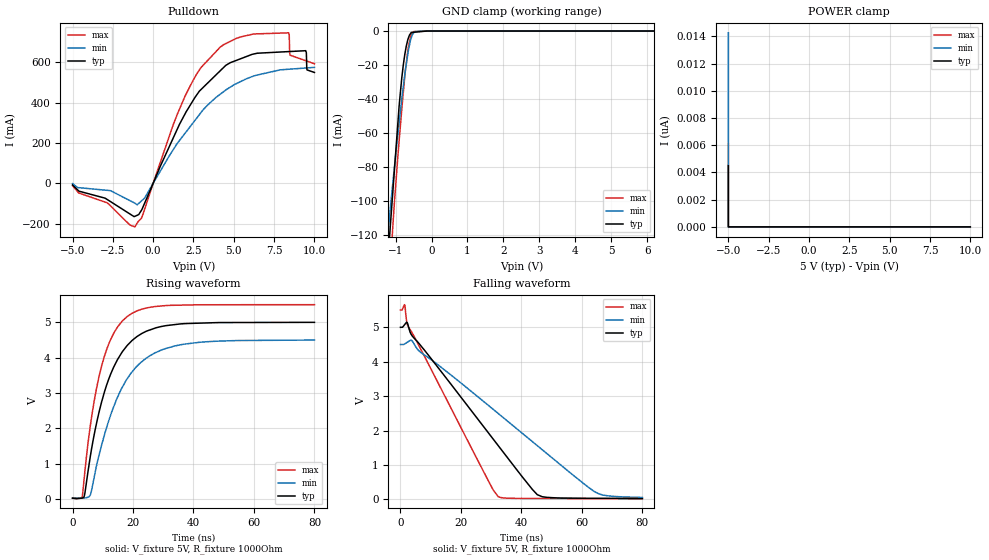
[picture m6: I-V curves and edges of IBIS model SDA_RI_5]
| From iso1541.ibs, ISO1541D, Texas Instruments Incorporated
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|   SDA Right 5V I/O Model
[Model]   SDA_RI_5
Model_type   I/O_open_drain
Polarity   Non-Inverting
Enable   Active-Low
Vinl = 1.35
Vinh = 3.85
Vmeas = 2.5
Vref = 2.5
Cref = 15pF
Rref = 1000
|   typ   min   max
|   (nom PVT)   (fast PVT)   (slow PVT)
C_comp   1.948p   1.600p   2.714p
|C_comp (ON state)   1.948p   1.600p   2.714p
|C_comp (OFF state)   3.853p   2.911p   4.851p
|PVT   Nom   Slow   Fast
[Voltage Range]   5   4.5   5.5
[Temperature Range]   27   136   -40
[Pullup Reference]   5   4.5   5.5
[Pulldown Reference]   -0   -0   -0
[Power Clamp Reference]   5   4.5   5.5
[GND Clamp Reference]   -0   -0   -0
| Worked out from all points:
|   slope of the pulldown table from 0 to 0.75 V, typ, clamps not added: 5.42 ohm
|   GND clamp passes 1 mA (typ) near -0.57 V on its own axis
|   falling waveform, V_fixture 5V, R_fixture 1000Ohm: 20-80 % time 26.2ns typ, 37ns min, 19.2ns max; typ from 5 V to 0.029 V
|   rising waveform, V_fixture 5V, R_fixture 1000Ohm: 20-80 % time 9.75ns typ, 11.9ns min, 7.57ns max; typ from 0.026 V to 5 V
[Pulldown]
|   Voltage   I(typ)   I(min)   I(max)
-5V       -8.402mA   -2.148mA   -12.24mA
-1.132V   -164.3mA   -99.13mA   -216.6mA
-722.2mV  -133.5mA   -87.59mA   -172.8mA
1.981V    345.2mA    248.6mA    433.2mA
4.155V    558.4mA    442mA      676mA
6.135V    640.1mA    529.7mA    739.6mA
8.4V      653.9mA    566.2mA    747mA
8.436V    654mA      566.4mA    736mA
8.483V    654.2mA    566.7mA    636.1mA
9.462V    658.2mA    572.4mA    608.5mA
9.538V    562.9mA    572.8mA    606.3mA
10V       550.1mA    575.5mA    593.3mA
[GND Clamp]
|   Voltage   I(typ)   I(min)   I(max)
-5V       -1.105A    -843.9mA   -1.313A
-1.288V   -159.8mA   -136.3mA   -194.2mA
-1.181V   -124.9mA   -112.2mA   -152.6mA
-1.132V   -110.8mA   -101.2mA   -133.6mA
-1.054V   -88.22mA   -84.78mA   -107.6mA
-899.1mV  -43.61mA   -53.84mA   -64.15mA
-828.5mV  -27.89mA   -40.2mA    -46.49mA
-743.6mV  -13.85mA   -25.7mA    -26.98mA
-645.7mV  -4.27mA    -11.69mA   -9.383mA
-563.5mV  -853uA     -4.012mA   -2.206mA
-252.8mV  -246.7uA   -2.576uA   -110.8uA
10V       0A         0A         0A
[POWER Clamp]
|   Voltage   I(typ)   I(min)   I(max)
-5V       4.495nA    14.27nA    6.141nA
-5V       0A         0A         0A
-5V       0A         0A         0A
10V       0A         0A         0A
[Ramp]
R_load = 1000
|   typ   min   max
dV/dt_r   2.98444/9.75768e-09   2.68036/1.18751e-08   3.28661/7.57239e-09
dV/dt_f   2.98239/2.61568e-08   2.66494/3.69956e-08   3.28605/1.91753e-08
[Falling Waveform]
V_fixture = 5V
V_fixture_min = 4.5V
V_fixture_max = 5.5V
R_fixture = 1000Ohm
C_fixture = 0F
|   Time   V(typ)   V(min)   V(max)
0s        5V         4.5V       5.5V
1.408ns   5.08V      4.518V     5.654V
2.504ns   5.069V     4.58V      5.03V
3.906ns   4.746V     4.6V       4.833V
6.652ns   4.474V     4.275V     4.376V
32.32ns   1.565V     2.499V     81.3mV
43.65ns   289.4mV    1.679V     29.22mV
46.85ns   80.77mV    1.447V     28.69mV
65.66ns   32.91mV    160mV      25.6mV
80ns      29.35mV    58.44mV    23.24mV
[Rising Waveform]
V_fixture = 5V
V_fixture_min = 4.5V
V_fixture_max = 5.5V
R_fixture = 1000Ohm
C_fixture = 0F
|   Time   V(typ)   V(min)   V(max)
0s        25.83mV    31.92mV    22.28mV
3.252ns   29.82mV    28.71mV    93.43mV
4.089ns   172.4mV    33.59mV    792.5mV
6.459ns   1.501V     316.2mV    2.411V
10.47ns   3.006V     1.791V     4.023V
13.66ns   3.742V     2.625V     4.699V
18.03ns   4.341V     3.398V     5.161V
25.73ns   4.789V     4.063V     5.427V
35.33ns   4.952V     4.359V     5.486V
80ns      5V         4.499V     5.5V
